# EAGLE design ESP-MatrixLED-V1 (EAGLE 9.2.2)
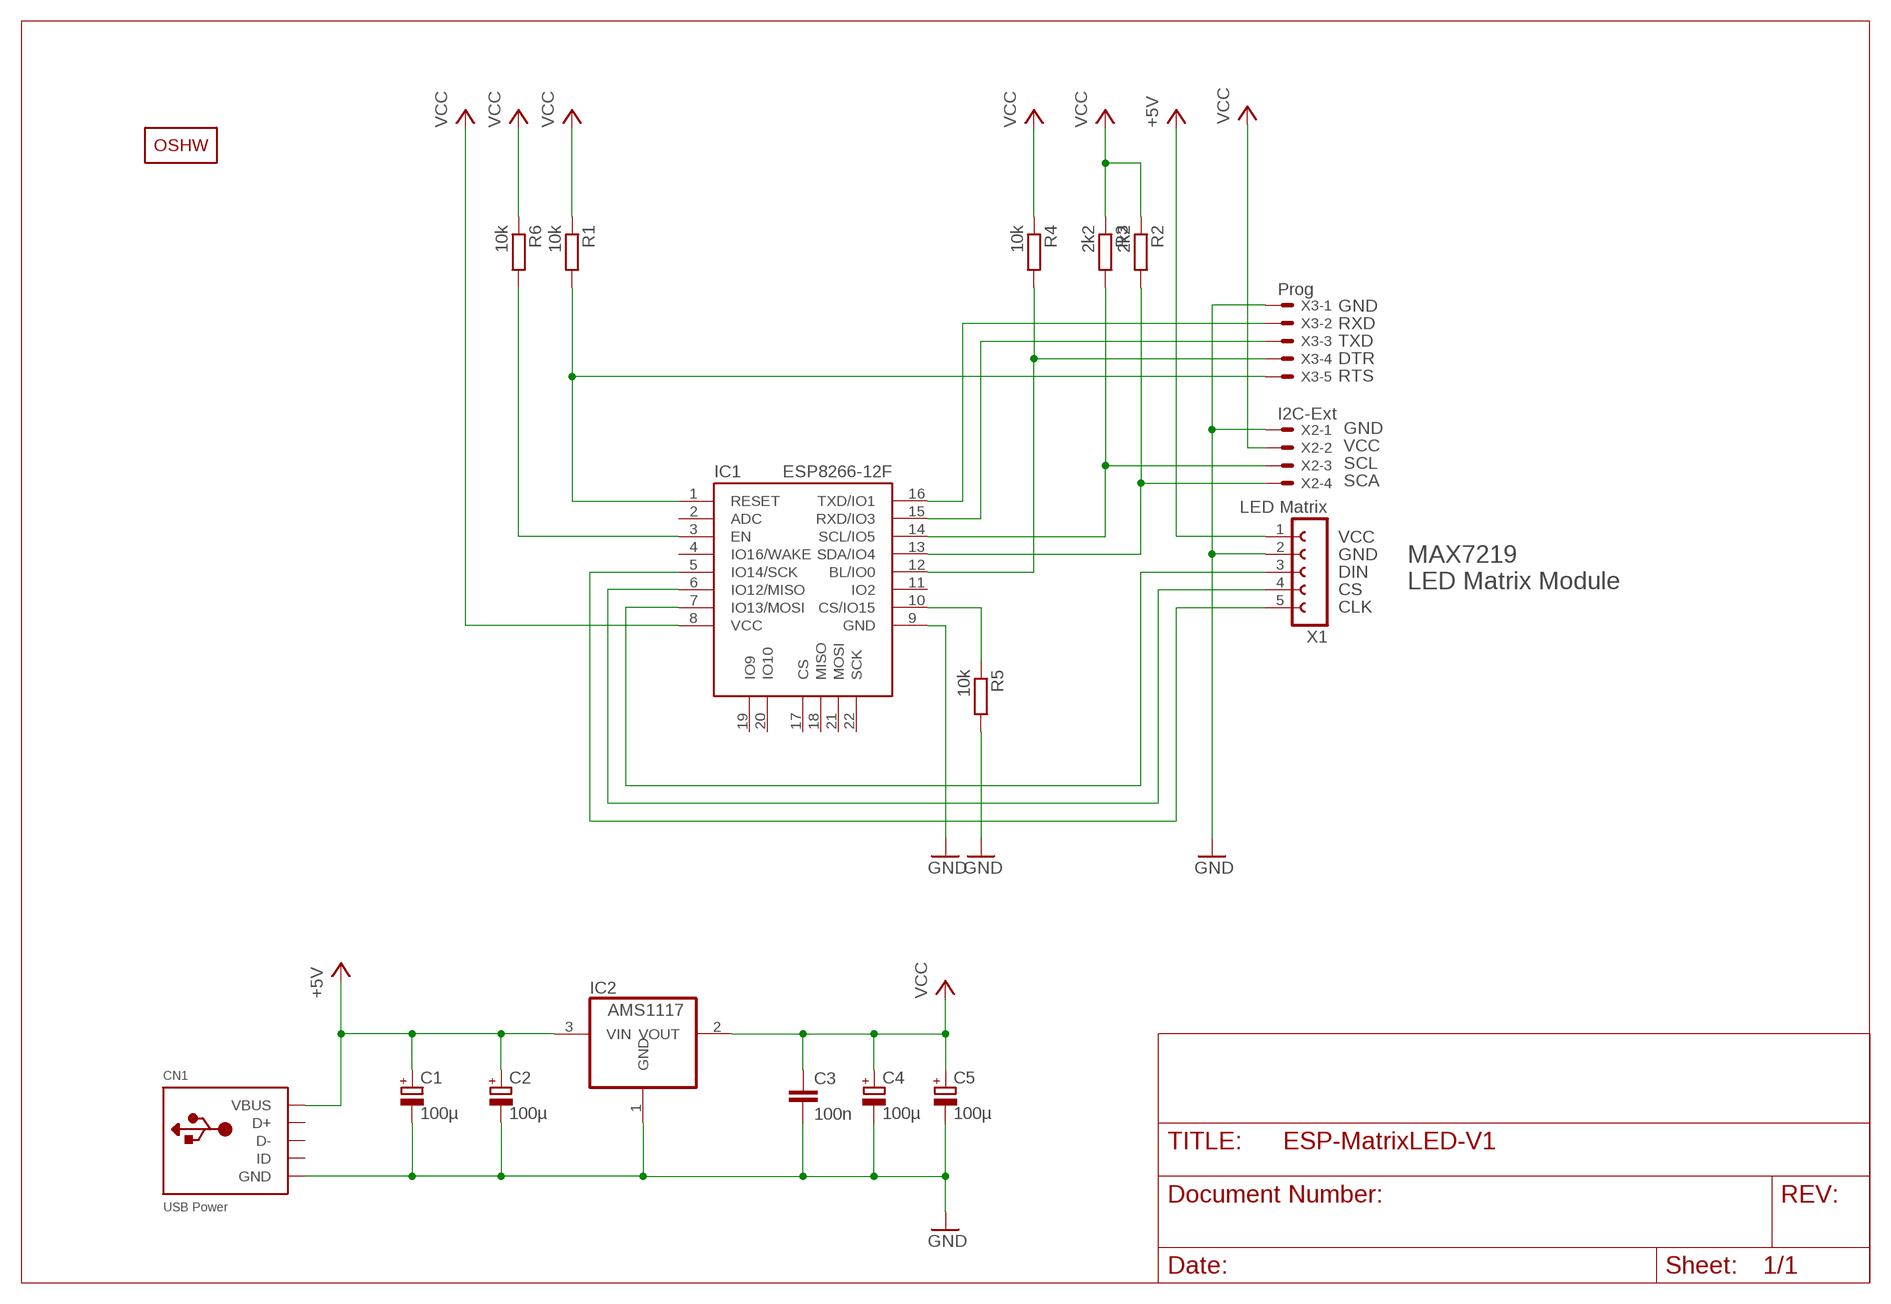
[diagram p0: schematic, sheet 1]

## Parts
C1  100µ  CPOL-EUCT7343  [CT7343]
C2  100µ  CPOL-EUCT7343  [CT7343]
C3  100n  C-EUC0603  [C0603]
C4  100µ  CPOL-EUCT7343  [CT7343]
C5  100µ  CPOL-EUCT7343  [CT7343]
CN1  USB Power  USBMINIB  [USB-MINIB]
IC1  ESP8266-12F  [ESP8266-12E]
IC2  AMS1117  REG1117SOT223  [SOT223]
LOGO1  OSHW_LOGOX0100  [OSHW_6X100]
R1  10k  R-EU_R0603  [R0603]
R2  2k2  R-EU_R0603  [R0603]
R3  2k2  R-EU_R0603  [R0603]
R4  10k  R-EU_R0603  [R0603]
R5  10k  R-EU_R0603  [R0603]
R6  10k  R-EU_R0603  [R0603]
X1  LED Matrix  FE05-1FE05-1  [FE05-1]
X2  I2C-Ext  JST-XH-04-PIN-LONG-PAD  [JST-XH-04-PACKAGE-LONG-PAD]
X3  Prog  JST-XH-05-PIN-SE  [JST-XH-05-PACKAGE-LONG-PAD-SE]

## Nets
+5V: C1.+ C2.+ CN1.VBUS IC2.3(VIN) X1.1
ESP_EN: IC1.3(EN) R6.2
ESP_PROG: IC1.12(BL/IO0) R4.2 X3.4
GND: C1.- C2.- C3.2 C4.- C5.- CN1.GND IC1.9(GND) IC2.1(GND) R5.2 X1.2 X2.1 X3.1
LED_CS: IC1.6(IO12/MISO) X1.4
LED_DIN: IC1.7(IO13/MOSI) X1.3
LED_SCK: IC1.5(IO14/SCK) X1.5
N$9: IC1.10(CS/IO15) R5.1
RESET: IC1.1(RESET) R1.2 X3.5
RXD: IC1.15(RXD/IO3) X3.3
SCL: IC1.14(SCL/IO5) R3.2 X2.3
SDA: IC1.13(SDA/IO4) R2.2 X2.4
TXD: IC1.16(TXD/IO1) X3.2
VCC: C3.1 C4.+ C5.+ IC1.8(VCC) IC2.2(VOUT) R1.1 R2.1 R3.1 R4.1 R6.1 X2.2
Unconnected: CN1.D+ CN1.D- CN1.ID IC1.2(ADC) IC1.4(IO16/WAKE) IC1.11(IO2) IC1.17(CS) IC1.18(MISO) IC1.19(IO9) IC1.20(IO10) IC1.21(MOSI) IC1.22(SCK)

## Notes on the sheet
- GND
  RXD
  TXD
  DTR
  RTS
- GND
  VCC
  SCL
  SCA
- MAX7219 
  LED Matrix Module
- VCC
  GND
  DIN
  CS
  CLK

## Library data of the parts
C1 C2 C4 C5 = rcl:CPOL-EU: POLARIZED CAPACITOR, European symbol; SPICEPREFIX: C
C3 = rcl:C-EU: CAPACITOR, European symbol; SPICEPREFIX: C
CN1 = microbuilder:USB: USB Connectors USBMINIB - Surface Mount Female Mini-B USB Connector 4UConnector: 06564
IC1 = we-chip:ESP8266-12F: AI-Thinker ESP-12F ESP8266 WiFi/WLAN-Module
IC2 = burr-brown:REG1117: 800mA and 1A Low Dropout (LDO) Positive Regulator 1.8V, 2.5V, 2.85V, 3.3V, 5V, and Adj
LOGO1 = we-symbol:OSHW_LOGO: Open-Source-Hardware Logo
R1-R6 = rcl:R-EU_: RESISTOR, European symbol; SPICEPREFIX: R
X1 = con-jojos:FE05-1: FEMALE HEADER
X2 = Rembrandt Electronics - JST XH Connectors v1-0:JST-XH-04-PIN: JST XH Connector 4 Pin Wire to board connector. Pitch: 2,54 mm, (0.100") Number of pins: 4 Created by Rembrandt Electronics www.rembrandtelectronics.com
X3 = Rembrandt Electronics - JST XH Connectors v1-0:JST-XH-05-PIN-SE: JST XH Connector 5 Pin Wire to board connector. Pitch: 2,54 mm, (0.100") Number of pins: 5 Created by Rembrandt Electronics www.rembrandtelectronics.com

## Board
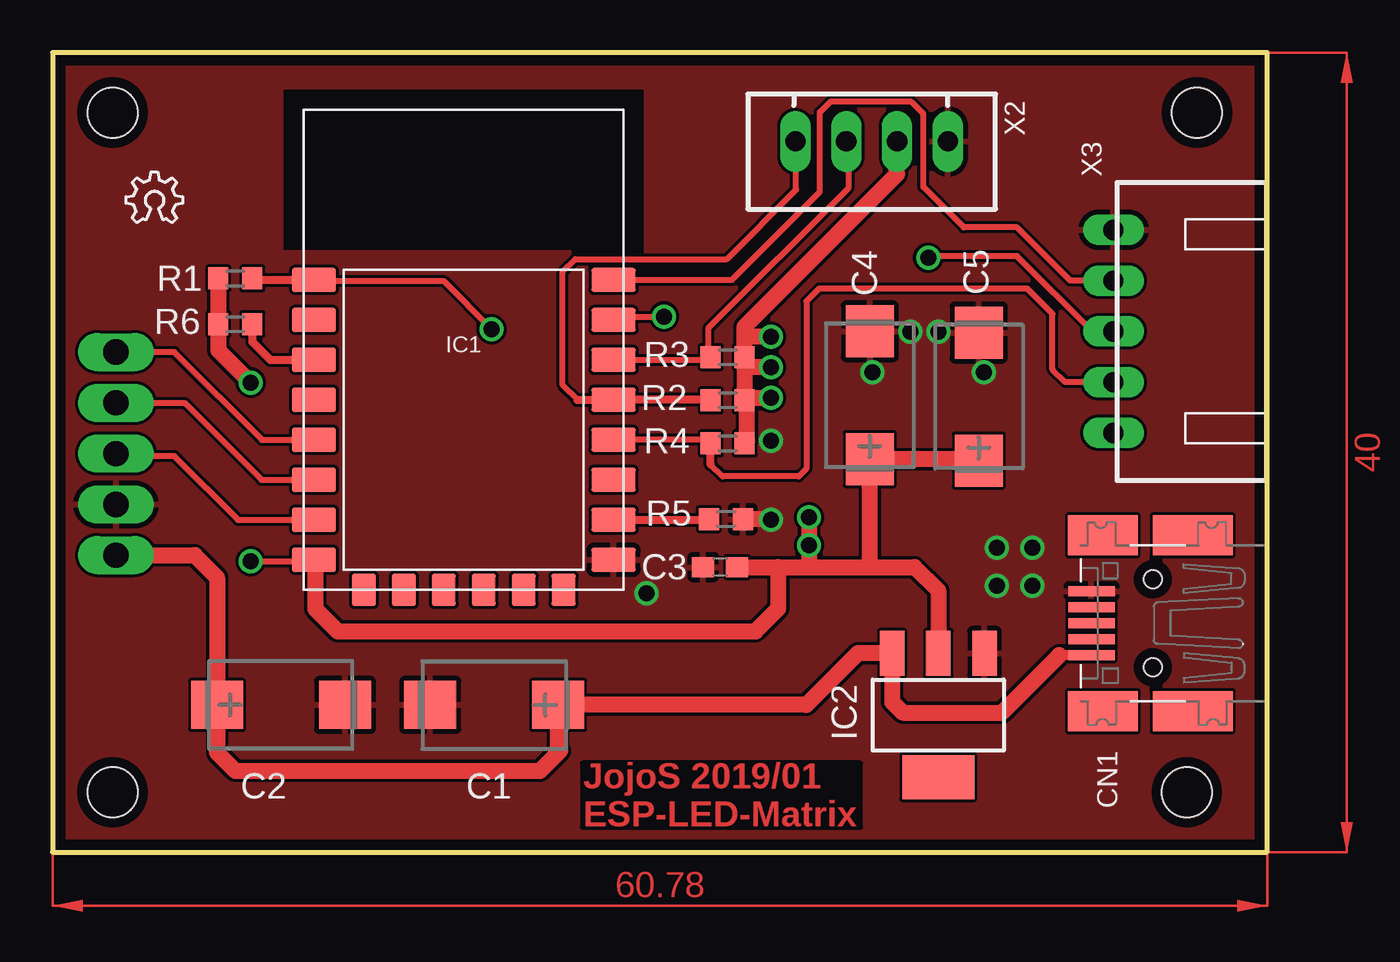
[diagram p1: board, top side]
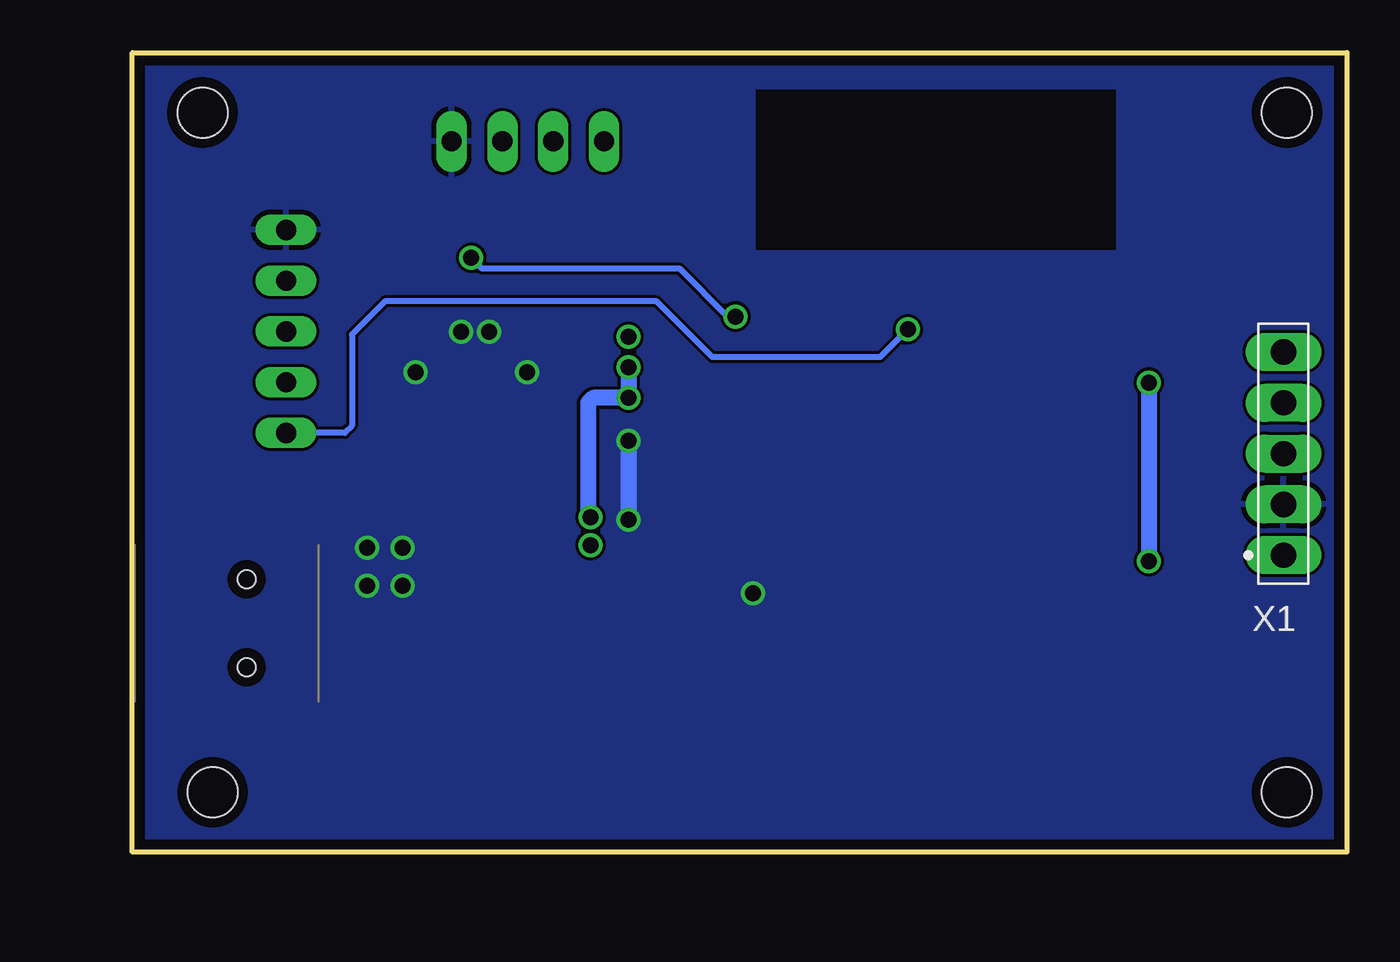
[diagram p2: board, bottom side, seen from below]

Size 60.78 x 40 mm. Coordinates in mm from the lower left corner, seen from the top.
Outline: 0,0 60.78,0 60.78,40 0,40 0,0
Copper layers (1*16): Top 0.035mm / dielectric 1.6mm / Bottom 0.035mm
Design rules "Elecrow_2-layer_PCB_eagle_rule": minimum track width 6mil, minimum drill 12mil, track to track 6mil, track to pad 6mil, pad to pad 6mil, via to via 8mil, smd to smd 0mil, copper to edge 20mil, drill to drill 10mil, minimum pad ring 6mil, minimum via ring 6mil, stop-mask expansion 0mil, vias tented up to drill 100mil, thermal gap 10mil
Holes 2.5 mm at 3,37 3,3 56.76,3 57.27,37

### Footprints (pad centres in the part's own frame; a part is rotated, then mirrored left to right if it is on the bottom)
CT7343 = smd 2.6 x 2.4: + -3.2,0; - 3.2,0
C0603 = smd 1.1 x 1: 1 -0.85,0; 2 0.85,0
USB-MINIB = smd 0.5 x 2.308: D+ 0,4.064; D- -0.8,4.064; GND 1.6,4.064; ID 0.8,4.064; VBUS -1.6,4.064 | smd 2 x 4: GND1 -4.4,-1; GND4 4.4,-1 | smd 2 x 3.5: GND2 -4.4,3.5; GND3 4.4,3.5 | hole 0.9: -2.2,1; 2.2,1
ESP8266-12E = smd 2.2 x 1.2: 1 -7.5,4.5; 2 -7.5,2.5; 3 -7.5,0.5; 4 -7.5,-1.5; 5 -7.5,-3.5; 6 -7.5,-5.5; 7 -7.5,-7.5; 8 -7.5,-9.5; 9 7.5,-9.5; 10 7.5,-7.5; 11 7.5,-5.5; 12 7.5,-3.5; 13 7.5,-1.5; 14 7.5,0.5; 15 7.5,2.5; 16 7.5,4.5 | smd 1.2 x 1.6: 17 -5,-11; 18 -3,-11; 19 -1,-11; 20 1,-11; 21 3,-11; 22 5,-11
SOT223 = smd 1.219 x 2.235: 1 -2.311,-3.099; 2 0,-3.099; 3 2.311,-3.099 | smd 3.6 x 2.2: 4 0,3.099
R0603 = smd 1 x 1.1: 1 -0.85,0; 2 0.85,0
FE05-1 = drill 1.261 pad 1.891 long: 1 0,0; 2 2.54,0; 3 5.08,0; 4 7.62,0; 5 10.16,0
JST-XH-04-PACKAGE-LONG-PAD = drill 1.016 long: 1 -3.81,0; 2 -1.27,0; 3 1.27,0; 4 3.81,0
JST-XH-05-PACKAGE-LONG-PAD-SE = drill 1.016 long: 1 -5.08,0; 2 -2.54,0; 3 0,0; 4 2.54,0; 5 5.08,0

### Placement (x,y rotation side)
C1  22.1,7.37 180 top
C2  11.43,7.37 0 top
C3  33.41,14.27 180 top
C4  40.89,22.86 90 top
C5  46.35,22.79 90 top
CN1  56.06,11.46 90 top
IC1  20.57,24.13 0 top
IC2  44.32,6.86 180 top
LOGO1  3.68,31.5 0 top
R1  9.14,28.7 0 top
R2  33.78,22.61 180 top
R3  33.78,24.77 180 top
R4  33.78,20.45 180 top
R5  33.7,16.67 0 top
R6  9.14,26.42 0 top
X1  3.17,14.86 90 bottom
X2  40.99,35.56 180 top
X3  53.09,26.05 270 top

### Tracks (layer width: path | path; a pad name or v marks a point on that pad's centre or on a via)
+5V
  Top 0.508: CN1.VBUS 50.37,9.86
  Top 0.813: X1.1 7.11,14.86 8.23,13.74 C2.+ 8.23,4.98 9.14,4.06 24.38,4.06 25.4,5.08 25.3,5.18 C1.+ 37.72,7.37 40.31,9.96 IC2.3 42.01,7.52 42.55,6.99 47.5,6.99 50.37,9.86
ESP_EN
  Top 0.406: R6.2 9.99,25.53 10.89,24.63 IC1.3
ESP_PROG
  Top 0.305: 32.93,19.39 33.53,18.8 37.34,18.8 37.72,19.18 37.72,27.56 38.35,28.19 48.77,28.19 50.04,26.92 50.04,24.15 50.67,23.51 X3.4 | 32.75,20.63 IC1.12
  Top 0.406: IC1.12 28.13,20.57 | 32.93,19.39 R4.2 32.75,20.63
GND  (via drill 0.8)
  Top 0.813: v35.94,16.64 35.91,16.67 R5.2
  Bottom 0.813: v35.94,20.57 v35.94,16.64
  other vias: 41.02,24 46.61,24 44.32,26.04 42.93,26.04 49.02,15.24 47.24,15.24 47.24,13.34 49.02,13.34 29.72,12.95
  pour Top: -0.51,40.26 -0.51,-0.51 61.21,-0.51 61.21,40.26
  pour Bottom: -0.25,40.13 61.21,40.13 61.21,-0.38 -0.25,-0.38
LED_CS
  Top 0.305: X1.4 6.6,22.48 10.45,18.63 IC1.6
LED_DIN
  Top 0.305: IC1.7 9.28,16.63 6.1,19.81 3.3,19.81
  Top 0.406: 3.3,19.81 X1.3
LED_SCK
  Top 0.305: IC1.5 10.48,20.63 6.1,25.02 X1.5
N$9
  Top 0.406: IC1.10 32.81,16.63 R5.1
RESET  (via drill 0.8)
  Top 0.305: IC1.1 13.13,28.57 19.56,28.57 v21.97,26.16
  Top 0.406: R1.2 10.07,28.63 IC1.1
  Bottom 0.305: v21.97,26.16 23.37,24.77 31.75,24.77 34.54,27.56 48.13,27.56 49.78,25.91 49.78,21.34 50.15,20.97 X3.5
RXD  (via drill 0.8)
  Top 0.305: v43.82,29.73 43.9,29.82 48.26,29.82 52.03,26.05 X3.3 | IC1.15 28.24,26.8 v30.61,26.8
  Bottom 0.305: v30.61,26.8 30.99,26.8 33.4,29.21 43.29,29.21 v43.82,29.73
SCL
  Top 0.305: X2.3 39.81,35.47 39.81,33.21 32.8,26.2 32.8,24.89 R3.2 32.8,24.63 IC1.14
SDA
  Top 0.305: 26.27,22.63 25.53,23.37 25.53,29.04 26.16,29.67 33.74,29.67 37.21,33.15 37.21,35.53
  Top 0.406: R2.2 32.91,22.63 IC1.13 26.27,22.63 | 37.21,35.53 X2.4
TXD
  Top 0.305: IC1.16 33.99,28.63 38.4,33.04 38.4,37.02 38.91,37.53 42.98,37.53 43.57,36.95 43.57,33.28 45.59,31.26 48.26,31.26 50.93,28.59 X3.2
VCC  (via drill 0.8)
  Top 0.305: v9.91,14.56 13.14,14.56
  Top 0.813: C5.+ 46.28,19.66 C4.+ 40.89,14.27 | R3.1 R2.1 34.76,22.73 | IC1.8 13.14,14.56 13.14,12.17 14.27,11.05 35.18,11.05 36.32,12.19 36.32,14.27 | R1.1 R6.1 8.29,25.11 v9.91,23.5 | 36.32,14.27 37.85,14.27 | 37.85,14.27 40.89,14.27 | 40.89,14.27 43.14,14.27 44.32,13.08 IC2.2 | R3.1 34.63,25.78 | 34.63,25.78 34.63,26.29 42.26,33.92 X2.2 | v35.94,24.26 34.63,24.26 R3.1 | 34.76,22.73 v35.94,22.73 | 37.85,14.27 v37.85,15.37 v37.85,16.76 | v35.94,25.78 34.63,25.78 | C3.1 36.32,14.27 | R4.1 34.76,20.57 34.76,22.73
  Bottom 0.813: v35.94,24.26 v35.94,22.73 37.72,22.73 37.97,22.48 37.97,16.89 v37.85,16.76 | v9.91,23.5 v9.91,14.56
(copper drawn outside any net)
  shapes: Top area x2

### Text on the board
Top: JojoS 2019/01 / ESP-LED-Matrix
